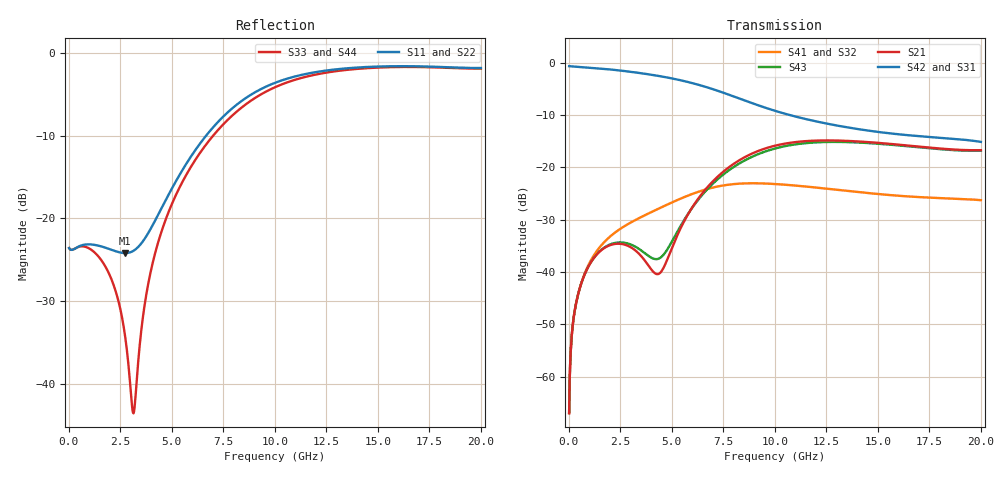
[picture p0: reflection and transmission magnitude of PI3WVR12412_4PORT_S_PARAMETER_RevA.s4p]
! NPort=4 DATA=800 NOISE=0 GROUPDELAY=0 COMPLEX_DATAFORMAT=POLAR
! NumOfBlock=1 NumOfParam=0
! .MODEL Smodel S TSTONEFILE=PI3WVR12412_4PORT_S_PARAMETER_RevA.s4p TYPE=S
!  -- The above .MODEL line can be used for the S element in the netlist.
! PORT DEFINITION
! PORT1 = INPUT+
! PORT2 = INPUT-
! PORT3 = OUTPUT+
! PORT4 = OUTPUT-
# Hz S MA R  50
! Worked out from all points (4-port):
!   800 points, 25 MHz to 20 GHz, reference 50 ohm
!   strongest paths, dB at 25 MHz, 5.025 GHz, 10.03 GHz, 15.03 GHz, 20 GHz:
!     S42: -0.6, -3.0, -9.2, -13.2, -15.1
!     S31: -0.6, -3.0, -9.2, -13.2, -15.1
!     S21: -66.9, -35.3, -15.8, -15.3, -16.7
!     S43: -66.9, -34.1, -16.4, -15.5, -16.8
!     S41: -67.0, -26.7, -23.2, -25.1, -26.3
!     S32: -67.0, -26.7, -23.2, -25.1, -26.3
!   lowest |S11| = -24.2 dB at 2.75 GHz (marker M1), VSWR 1.13, Z = 45 - j3.13 ohm
!   |S11| at or under -10 dB: start of sweep to 6.664 GHz
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2.5e7  0.06619 -2.3  0.0004498 87.2  0.9283 -0.6  0.0004469 87.2
       0.0004498 87.2  0.06619 -2.3  0.0004469 87.2  0.9283 -0.6
       0.9283 -0.6  0.0004469 87.2  0.06625 -1.9  0.0004498 87.3
       0.0004469 87.2  0.9283 -0.6  0.0004498 87.3  0.06625 -1.9
7.25e8  0.06925 -32.1  0.008941 68.5  0.9063 -14.3  0.009077 67.1
        0.008941 68.5  0.06925 -32.1  0.009077 67.1  0.9063 -14.3
        0.9063 -14.3  0.009078 67.1  0.06771 -19.9  0.008946 69.4
        0.009078 67.1  0.9063 -14.3  0.008946 69.4  0.06771 -19.9
2.75e9  0.06172 -145.9  0.01821 41.9  0.832 -50.9  0.02776 35.3
        0.01821 41.9  0.06172 -145.9  0.02776 35.3  0.832 -50.9
        0.8321 -50.9  0.02777 35.3  0.01904 -97.5  0.019 46.5
        0.02777 35.3  0.8321 -50.9  0.019 46.5  0.01904 -97.5
3.15e9  0.06379 -173.2  0.0166 40.0  0.8132 -57.9  0.03076 29.8
        0.0166 40.0  0.06379 -173.2  0.03076 29.8  0.8132 -57.9
        0.8132 -57.9  0.03076 29.8  0.006624 179.6  0.01785 45.8
        0.03076 29.8  0.8132 -57.9  0.01785 45.8  0.006624 179.6
4.7e9  0.1283 97.6  0.01202 108.9  0.7286 -85.0  0.04335 9.6
       0.01202 108.9  0.1283 97.6  0.04335 9.6  0.7286 -85.0
       0.7287 -85.0  0.04335 9.7  0.09775 61.2  0.01549 96.8
       0.04335 9.7  0.7287 -85.0  0.01549 96.8  0.09775 61.2
8.525e9  0.5279 -5.5  0.1248 90.7  0.4376 -145.2  0.07034 -58.5
         0.1248 90.7  0.5279 -5.5  0.07034 -58.5  0.4376 -145.2
         0.4377 -145.1  0.07036 -58.5  0.4827 -11.8  0.1161 87.3
         0.07036 -58.5  0.4377 -145.1  0.1161 87.3  0.4827 -11.8
2e10  0.8131 -106.6  0.1462 -2.5  0.1753 93.8  0.04861 135.2
      0.1462 -2.5  0.8131 -106.6  0.04861 135.2  0.1753 93.8
      0.1754 93.8  0.04865 135.2  0.806 -106.8  0.1445 -2.0
      0.04865 135.2  0.1754 93.8  0.1445 -2.0  0.806 -106.8
